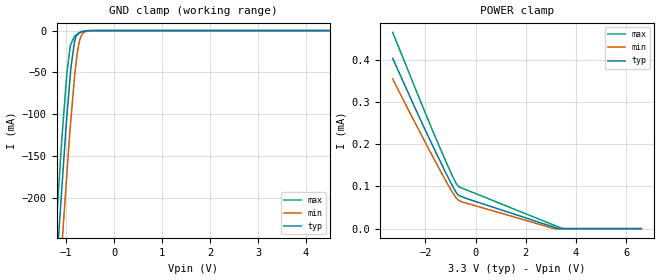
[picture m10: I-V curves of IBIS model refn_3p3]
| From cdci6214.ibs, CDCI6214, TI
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|   refn_3p3 Model
[Model]   refn_3p3
Model_type   Input
Vinl = 0.66
Vinh = 2.64
|   typ   min   max
C_comp   7.404E-13   6.960E-13   7.875E-13
|  Where Nom  PVT is Nominal Process, 3.3V,   32C
|   Fast PVT is Strong Process,  3.465V, -35C
|   Slow PVT is Weak Process,   3.135V,  110C
[Model spec]
|subparameter
Vinl   0.66   0.627   0.693
Vinh   2.64   2.508   2.772
[Voltage Range]   3.3   3.135   3.465
|Junction Temperature
[Temperature Range]   32   110   -35
[Power Clamp Reference]   3.3   3.135   3.465
[GND Clamp Reference]   0   0   0
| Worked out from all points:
|   GND clamp passes 1 mA (typ) near -0.65 V on its own axis
[GND Clamp]
|   Voltage   I(typ)   I(min)   I(max)
-3.3V     -2.319A    -2.382A    -2.268A
-1.236V   -318.5mA   -389.4mA   -258.8mA
-1.146V   -236.1mA   -309.3mA   -179.3mA
-1.087V   -186.9mA   -257.5mA   -127.8mA
-1.055V   -159.9mA   -229mA     -103.9mA
-982.4mV  -101.3mA   -169.9mA   -49.77mA
-901.4mV  -45.1mA    -107.1mA   -16.34mA
-794.8mV  -7.455mA   -39.14mA   -5.586mA
-741.3mV  -3.111mA   -17.94mA   -3.782mA
-683.6mV  -1.279mA   -6.213mA   -1.832mA
-348.3mV  -7.821uA   -9.932uA   -8.697uA
6.6V      0A         0A         0A
[POWER Clamp]
|   Voltage   I(typ)   I(min)   I(max)
-3.3V     402.8uA    354.3uA    464.2uA
-2.481V   294.7uA    258.6uA    343.6uA
-1.481V   168.2uA    145.5uA    199.8uA
-955.6mV  105.1uA    89.18uA    128.8uA
-763.6mV  85.12uA    72.1uA     106.1uA
-672.5mV  78.89uA    66.91uA    99.61uA
-400.4mV  72.06uA    60.89uA    92.58uA
3.134V    3.239uA    11.31nA    7.941uA
3.299V    1.655nA    0A         3.965uA
3.464V    0A         0A         17.1nA
6.6V      0A         0A         0A
